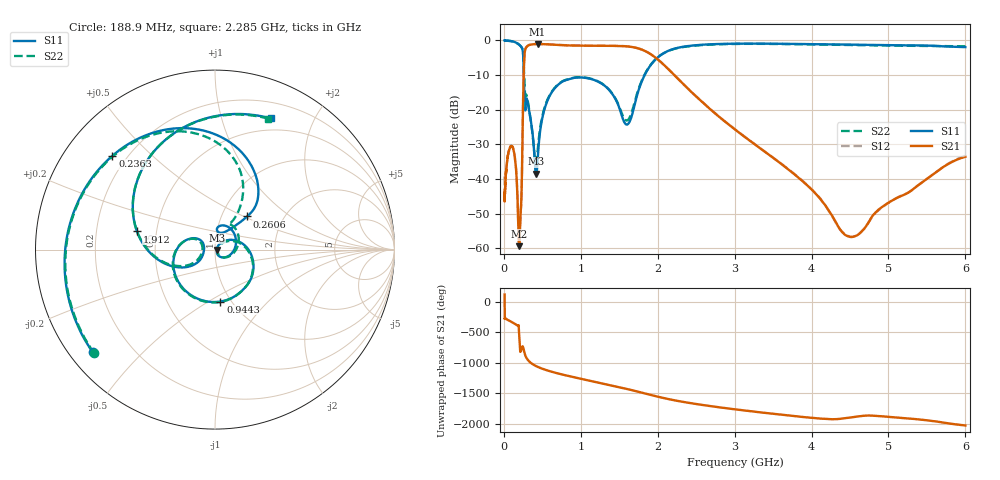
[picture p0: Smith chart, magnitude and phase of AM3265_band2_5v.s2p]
!Agilent Technologies,E8364B,MY43040894,A.07.50.67
!Agilent E8364B: A.07.50.67
!Date: Friday, May 09, 2025 07:24:44
!Correction: S11(Full 2 Port(1,2))
!S21(Full 2 Port(1,2))
!S12(Full 2 Port(1,2))
!S22(Full 2 Port(1,2))
!S2P File: Measurements: S11, S21, S12, S22:Log Frequency Sweep
# Hz S  dB  R 50
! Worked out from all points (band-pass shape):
!   3201 points, 10 MHz to 6 GHz, reference 50 ohm
!   highest |S21| = -1.04 dB at 439.1 MHz (marker M1); lowest = -59.4 dB at 200.6 MHz (marker M2)
!   |S21| within 3 dB of the highest: 269.4 MHz to 1.914 GHz (1.644 GHz wide, 151 % of centre)
!   lowest |S11| = -38.5 dB at 419.4 MHz (marker M3), VSWR 1.02, Z = 51.2 - j0.187 ohm
!   |S11| at or under -10 dB: 259 MHz to 1.83 GHz (1.571 GHz wide, 150 % of centre)
!   |S22| runs from -35.5 to 0.0 dB; largest |S21 - S12| = 0.012
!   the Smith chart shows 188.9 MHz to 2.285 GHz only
!   S11 on the Smith chart (normalised r, x): 188.9 MHz: 0.07, -0.36; 236.3 MHz: 0.15, +0.38; 260.6 MHz: 1.32, +0.52; 944.3 MHz: 0.89, -0.56; 1.912 GHz: 0.39, +0.10; 2.285 GHz: 0.37, +1.45
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1e7  0.00 -6.0  -44.92 116.2  -39.29 82.7  -0.08 -5.6
2.908064e7  -0.04 -16.8  -37.89 75.3  -37.86 75.0  -0.04 -16.8
8.439949e7  -0.13 -50.4  -30.81 39.1  -30.67 38.6  -0.17 -50.7
1.888919e8  -1.02 -139.9  -54.31 -31.8  -54.42 12.5  -1.05 -139.4
2.005665e8  -1.22 -155.1  -59.40 150.6  -59.02 -162.8  -1.25 -154.3
2.362917e8  -2.22 137.5  -37.48 -26.3  -37.39 -28.0  -2.18 141.9
2.44949e8  -2.92 109.6  -24.73 -12.2  -24.74 -12.2  -2.82 116.8
2.606087e8  -11.79 45.8  -8.01 -76.0  -7.98 -76.0  -8.69 64.7
2.920618e8  -16.77 66.2  -1.97 163.1  -1.93 163.0  -15.66 50.2
4.19386e8  -38.46 -8.8  -1.04 24.3  -1.00 24.3  -35.44 -0.3
4.391187e8  -34.83 42.0  -1.04 12.5  -1.00 12.5  -32.00 34.5
7.123273e8  -12.67 -22.8  -1.29 -98.7  -1.26 -98.7  -12.55 -26.3
9.442607e8  -10.73 -84.1  -1.47 -167.3  -1.44 -167.3  -10.63 -86.7
1.342426e9  -13.68 177.0  -1.54 84.1  -1.51 84.1  -13.62 176.8
1.912303e9  -7.01 166.9  -4.02 -89.0  -3.98 -89.0  -6.93 166.0
2.067357e9  -3.81 121.6  -6.77 -136.1  -6.74 -136.0  -3.82 121.9
2.284673e9  -2.00 67.1  -11.56 168.3  -11.54 168.3  -2.07 67.9
3.202913e9  -0.90 -91.4  -29.03 6.0  -29.01 6.2  -0.97 -91.5
3.818953e9  -1.01 -178.2  -39.42 -80.4  -39.30 -80.5  -1.09 -179.7
4.490206e9  -1.21 92.0  -56.66 -100.9  -56.64 -99.6  -1.30 90.5
5.185309e9  -1.41 1.2  -44.73 -108.1  -44.67 -108.3  -1.52 1.3
6e9  -1.93 -97.0  -33.58 132.3  -33.36 131.3  -1.68 -96.5
